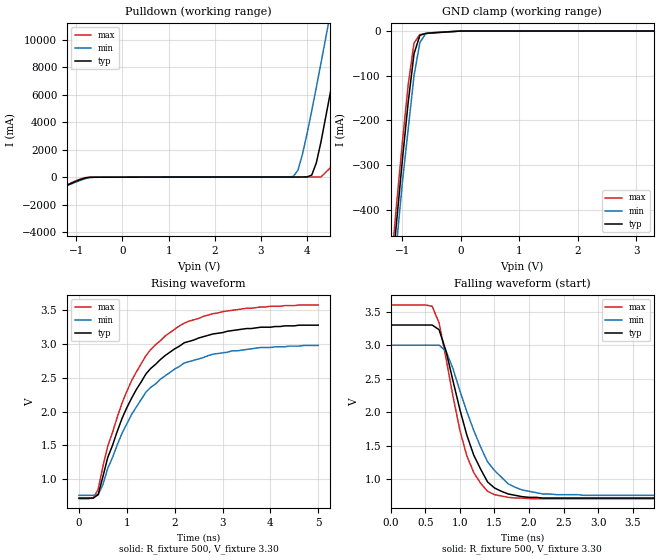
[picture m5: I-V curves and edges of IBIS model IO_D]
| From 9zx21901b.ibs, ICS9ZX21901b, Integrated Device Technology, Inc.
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|   Model IO_D
[Model]   IO_D
Model_type   I/O_open_drain
Polarity   Non-Inverting
Enable   Active-High
Vinl =   1.00V
Vinh =   2.00V
Vmeas =   0.350V
Cref =   2.00pF
Rref =   0.000
Vref =   0.350V
C_comp   3.40pF   2.85pF   3.95pF
[Temperature Range]   27.00   70.00   0.000
[Voltage Range]   3.30V   3.00V   3.60V
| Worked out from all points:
|   slope of the pulldown table from 0 to 0.495 V, typ, clamps not added: 131 ohm
|   GND clamp passes 1 mA (typ) near -0.12 V on its own axis
|   rising waveform, R_fixture 500, V_fixture 3.30: 20-80 % time 1.13ns typ, 1.18ns min, 1.1ns max; typ from 0.72 V to 3.28 V
|   falling waveform, R_fixture 500, V_fixture 3.30: 20-80 % time 430ps typ, 510ps min, 367ps max; typ from 3.3 V to 0.72 V
[Pulldown]
| voltage   I(typ)   I(min)   I(max)
-3.3V     -3.78A     -3.65A     -3.87A
-800mV    -50.99mA   -100mA     -26.91mA
3.7V      9.44mA     53.55mA    11.23mA
3.8V      10.07mA    490mA      11.25mA
3.9V      12.32mA    1.67A      11.27mA
4.1V      150mA      4.83A      11.65mA
4.3V      2.56A      8.29A      17.33mA
4.5V      6.09A      11.85A     670mA
4.7V      9.81A      15.47A     3.91A
4.9V      13.62A     19.11A     7.69A
5.1V      17.46A     22.78A     11.6A
6.6V      46.76A     50.55A     41.81A
[GND_clamp]
| voltage   I(typ)   I(min)   I(max)
-3.3V     -3.78A     -3.65A     -3.87A
-1.2V     -570mA     -610mA     -540mA
-1.1V     -430mA     -480mA     -390mA
-1V       -290mA     -340mA     -250mA
-900mV    -160mA     -220mA     -120mA
-800mV    -50.99mA   -100mA     -26.91mA
-700mV    -9.68mA    -25.77mA   -7.84mA
-600mV    -5.33mA    -5.93mA    -5.63mA
0V        0A         0A         0A
3.3V      150pA      220pA      150pA
[Ramp]
| variable   typ   min   max
dV/dt_r   1.54/1.11n   1.33/1.16n   1.72/1.07n
dV/dt_f   1.55/0.42n   1.34/0.53n   1.73/0.36n
R_load = 500
[Rising Waveform]
R_fixture = 500
V_fixture = 3.30
V_fixture_min = 3.00
V_fixture_max = 3.60
| time   V(typ)   V(min)   V(max)
0s        720mV      760mV      710mV
300ps     720mV      760mV      720mV
400ps     770mV      770mV      850mV
600ps     1.32V      1.16V      1.49V
1ns       2.06V      1.82V      2.3V
1.4ns     2.56V      2.29V      2.83V
1.8ns     2.83V      2.53V      3.12V
2.2ns     3.02V      2.72V      3.31V
3ns       3.17V      2.87V      3.48V
5ns       3.28V      2.98V      3.58V
[Falling Waveform]
R_fixture = 500
V_fixture = 3.30
V_fixture_min = 3.00
V_fixture_max = 3.60
| time   V(typ)   V(min)   V(max)
0s        3.3V       3V         3.6V
600ps     3.3V       3V         3.58V
700ps     3.23V      3V         3.33V
800ps     2.91V      2.91V      2.8V
1ns       2.04V      2.32V      1.73V
1.1ns     1.66V      2.01V      1.35V
1.4ns     960mV      1.26V      820mV
1.7ns     780mV      930mV      730mV
2.2ns     720mV      780mV      710mV
5ns       720mV      760mV      710mV
